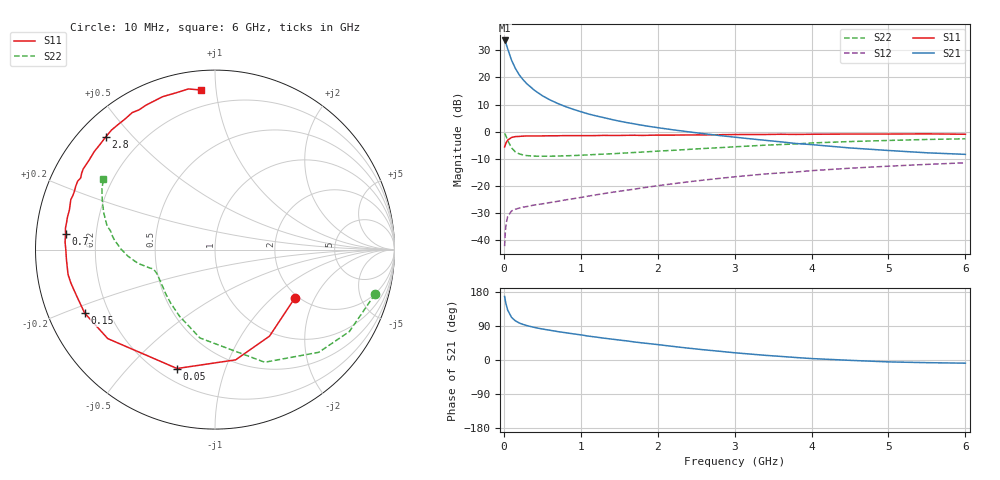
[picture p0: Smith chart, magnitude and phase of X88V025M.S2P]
! SIEMENS Small Signal Semiconductors
! BFP136W
! Si NPN RF Bipolar Junction Transistor in SOT343
! VCE = 8 V  IC = 25 mA
! Common Emitter S-Parameters:  September  1994
# GHz  S  MA  R  50
!  f  S11  S21  S12  S22
! GHz  MAG  ANG  MAG  ANG  MAG  ANG  MAG  ANG
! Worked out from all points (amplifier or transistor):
!   40 points, 10 MHz to 6 GHz, reference 50 ohm
!   highest |S21| = 33.7 dB at 10 MHz (marker M1)
!   |S21| within 3 dB of that: start of sweep to 48.76 MHz
!   unconditionally stable (mu >= 1): 900.6 MHz to 2.839 GHz
!   at 200 MHz: K = 0.37, MSG = 24.6 dB, |S12| = -28.3 dB
!   at 1.5 GHz: K = 1.14, MAG = 10.7 dB, |S12| = -22.1 dB
!   at 6 GHz: K = 0.96, MSG = 1.6 dB, |S12| = -11.5 dB
!   S11 on the Smith chart (normalised r, x): 10 MHz: 1.91, -1.42; 50 MHz: 0.27, -0.69; 150 MHz: 0.11, -0.23; 700 MHz: 0.09, +0.05; 2.8 GHz: 0.08, +0.42; 6 GHz: 0.10, +0.91
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0.01  0.5202 -31.3  48.41 167.7  0.0076 76.6  0.9253 -15.6
0.02  0.5699 -57.8  45.03 156.2  0.0144 67.2  0.8767 -31.4
0.03  0.6249 -79.4  41.8 146.6  0.0199 59.6  0.8134 -44.7
0.05  0.6954 -107.7  33.83 131.6  0.0269 46.2  0.6859 -66.2
0.1  0.7764 -140.3  20.97 112.5  0.0341 32.6  0.4996 -99.6
0.15  0.8078 -154.0  14.73 103.3  0.0366 28.6  0.4206 -118.0
0.2  0.8131 -161.6  11.22 97.7  0.0385 27.0  0.3868 -129.8
0.25  0.8242 -166.9  9.103 93.8  0.04 27.3  0.3697 -137.7
0.3  0.8304 -170.4  7.637 90.8  0.0411 27.6  0.3592 -143.2
0.4  0.8295 -176.2  5.771 85.8  0.044 29.7  0.3515 -150.4
0.5  0.8311 -179.9  4.609 81.8  0.046 31.9  0.3497 -155.1
0.6  0.8364 177.1  3.848 78.5  0.0487 34.0  0.3505 -157.8
0.7  0.837 174.0  3.313 75.0  0.0513 36.8  0.3532 -159.5
0.9  0.8406 169.6  2.588 69.1  0.0573 40.6  0.3598 -162.2
1.1  0.8408 164.8  2.115 63.0  0.0641 43.9  0.371 -163.7
1.5  0.8473 157.9  1.559 52.7  0.0787 48.5  0.3958 -166.1
2.2  0.8603 144.9  1.077 35.8  0.1083 50.2  0.4499 -171.6
2.8  0.8744 134.1  0.846 23.1  0.1361 48.3  0.5034 -178.0
3.2  0.8816 127.5  0.736 15.7  0.1547 45.8  0.5405 177.3
4.5  0.9006 108.9  0.498 -0.9  0.2101 36.1  0.6537 161.6
5.5  0.9073 99.4  0.405 -7.0  0.2472 27.6  0.7147 151.8
6  0.8922 94.9  0.379 -8.4  0.2648 23.2  0.7353 147.7
